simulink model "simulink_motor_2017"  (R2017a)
settings: Solver=VariableStepAuto  StartTime=0.0  StopTime=1  MaxStep=0.0001  RelTol=1e-5
undefined symbols (not defined in the file or in its folder): j

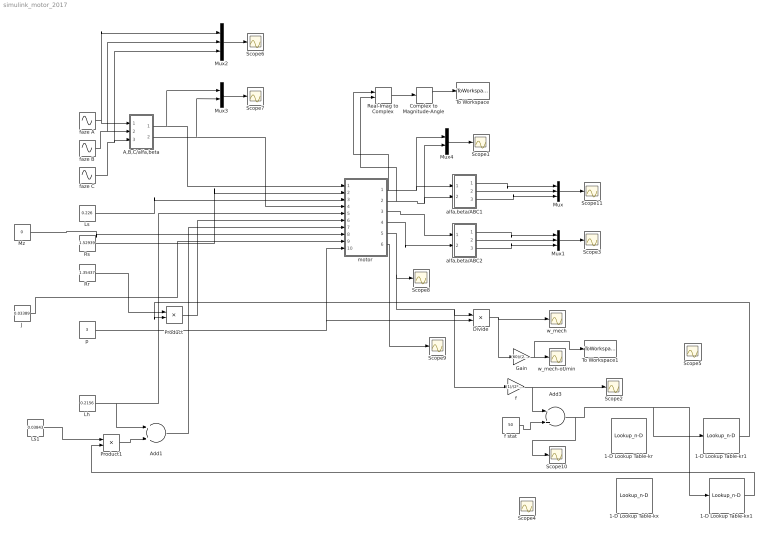
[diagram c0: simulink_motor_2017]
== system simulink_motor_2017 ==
  1-D Lookup Table-kr : Lookup_n-D  NumberOfTableDimensions=1  BreakpointsForDimension1="[0\t0.505050505050505\t1.01010101010101\t1.51515151515152\t2.02020202020202\t2.52525252525253\t3.03030303030303\t3.53535353535354\t4.04040404040404\t4.54545454545455\t5.05050505050505\t5.55555555555556\t6.06060606060606\t6.56565656565657\t7.07070707070707\t7.57575757575758\t8.08080808080808\t8.58585858585859\t9.09090909090909\t9.59595959595960\t10.1010101010101\t10.6060606060606\t11.1111111111111\t11.6161616161616\t12.12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"  Table="[1.00000000000000\t1.00008864994525\t1.00035453875263\t1.00079748344328\t1.00141717940610\t1.00221320092722\t1.00318500192865\t1.00433191691399\t1.00565316211802\t1.00714783685648\t1.00881492507177\t1.01065329706958\t1.01266171144098\t1.01483881716387\t1.01718315587736\t1.01969316432170\t1.02236717693666\t1.02520342860997\t1.02820005756793\t1.03135510839921\t1.03466653520308\t1.03813220485274\t1.04174990036446\t1.045517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"  InternalRulePriority=Speed  RndMeth=Simplest
  1-D Lookup Table-kr1 : Lookup_n-D  NumberOfTableDimensions=1  BreakpointsForDimension1="[0\t1.02040816326531\t2.04081632653061\t3.06122448979592\t4.08163265306123\t5.10204081632653\t6.12244897959184\t7.14285714285714\t8.16326530612245\t9.18367346938776\t10.2040816326531\t11.2244897959184\t12.2448979591837\t13.2653061224490\t14.2857142857143\t15.3061224489796\t16.3265306122449\t17.3469387755102\t18.3673469387755\t19.3877551020408\t20.4081632653061\t21.4285714285714\t22.4489795918367\t23.4693877551020\t24.489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"  Table="[1.00000000000000\t1.00077060964083\t1.00307777507260\t1.00690757634345\t1.01223704661737\t1.01903451494662\t1.02726007276191\t1.03686615140433\t1.04779819537135\t1.05999541393792\t1.07339159250137\t1.08791594439901\t1.10349398404126\t1.12004840293262\t1.13749993143670\t1.15576817087600\t1.17477238262788\t1.19443222316750\t1.21466841640173\t1.23540335703097\t1.25656164097697\t1.27807052105181\t1.29986028795912\t1.321864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"  InternalRulePriority=Speed  RndMeth=Simplest
  1-D Lookup Table-kx : Lookup_n-D  NumberOfTableDimensions=1  BreakpointsForDimension1="[0\t0.505050505050505\t1.01010101010101\t1.51515151515152\t2.02020202020202\t2.52525252525253\t3.03030303030303\t3.53535353535354\t4.04040404040404\t4.54545454545455\t5.05050505050505\t5.55555555555556\t6.06060606060606\t6.56565656565657\t7.07070707070707\t7.57575757575758\t8.08080808080808\t8.58585858585859\t9.09090909090909\t9.59595959595960\t10.1010101010101\t10.6060606060606\t11.1111111111111\t11.6161616161616\t12.12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"  Table="[1.04727985024947\t1.04725773631299\t1.04719140989840\t1.04708091716353\t1.04692633494882\t1.04672777064382\t1.04648536200084\t1.04619927689636\t1.04586971304107\t1.04549689763934\t1.04508108699933\t1.04462256609487\t1.04412164808060\t1.04357867376190\t1.04299401102106\t1.04236805420188\t1.04170122345412\t1.04099396404022\t1.04024674560607\t1.03946006141828\t1.03863442756993\t1.03777038215741\t1.03686848443050\t1.035929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"  InternalRulePriority=Speed  RndMeth=Simplest
  1-D Lookup Table-kx1 : Lookup_n-D  NumberOfTableDimensions=1  BreakpointsForDimension1="[0\t1.02040816326531\t2.04081632653061\t3.06122448979592\t4.08163265306123\t5.10204081632653\t6.12244897959184\t7.14285714285714\t8.16326530612245\t9.18367346938776\t10.2040816326531\t11.2244897959184\t12.2448979591837\t13.2653061224490\t14.2857142857143\t15.3061224489796\t16.3265306122449\t17.3469387755102\t18.3673469387755\t19.3877551020408\t20.4081632653061\t21.4285714285714\t22.4489795918367\t23.4693877551020\t24.489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"  Table="[1.00000000000000\t0.999555176608620\t0.998223403700545\t0.996012732286468\t0.992936445906495\t0.989012862377403\t0.984265063983984\t0.978720563445998\t0.972410914526099\t0.965371277307041\t0.957639948925946\t0.949257870899851\t0.940268124122870\t0.930715422193039\t0.920645612984507\t0.910105197377543\t0.899140872861085\t0.887799108398502\t0.876125755562974\t0.864165699565028\t0.851962552463579\t0.839558389616062\t0.82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"  InternalRulePriority=Speed  RndMeth=Simplest
  A,B,C/alfa,beta : Subsystem
  Add1 : Sum
  Add3 : Sum  Inputs=-+
  Complex to Magnitude-Angle : ComplexToMagnitudeAngle
  Divide : Product  Inputs=*/
  Gain : Gain  Gain=(60)/(2*pi)
  J : Constant  Value=0.03389
  Lh : Constant  Value=0.2156
  Ls : Constant  Value=0.226
  Ls1 : Constant  Value=0.03843
  Mux : Mux  Inputs=3
  Mux1 : Mux  Inputs=3
  Mux2 : Mux  Inputs=3
  Mux3 : Mux  Inputs=2
  Mux4 : Mux  Inputs=2
  Mz : Constant  Value=0
  Product : Product
  Product1 : Product
  Real-Imag to Complex : RealImagToComplex
  Rr : Constant  Value=1.35437
  Rs : Constant  Value=1.52939
  Scope{1..11} (11 alike) : Scope
  To Workspace : ToWorkspace  VariableName=Istat  SampleTime=-1
  To Workspace1 : ToWorkspace  VariableName=ot  SampleTime=-1
  alfa,beta/ABC1 : Subsystem
  alfa,beta/ABC2 : Subsystem
  f : Gain  Gain=(1)/(2*pi)
  f stat : Constant  Value=50
  faze A : Sin  Amplitude=230*1.41421356237309  Frequency=314.159265  SampleTime=0
  faze B : Sin  Amplitude=230*1.41421356237309  Frequency=314.159265  Phase=-(2*pi/3)  SampleTime=0
  faze C : Sin  Amplitude=230*1.41421356237309  Frequency=314.159265  Phase=(2*pi/3)  SampleTime=0
  motor : Subsystem
  p : Constant  Value=3
  w_mech : Scope
  w_mech-ot/min : Scope
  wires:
  faze A/1 -> Mux2/1, A,B,C/alfa,beta/1(In1)
  faze B/1 -> Mux2/2, A,B,C/alfa,beta/2(In2)
  faze C/1 -> Mux2/3, A,B,C/alfa,beta/3(In3)
  A,B,C/alfa,beta/1(Out1) -> Mux3/1, motor/1(Us_alfa)
  Rs/1 -> motor/2(Rs)
  Ls/1 -> motor/3(Ls)
  Lh/1 -> Add1/1, motor/5(Lh)
  motor/3(Ir_alfa1) -> alfa,beta/ABC2/1(Ir_alfa)
  motor/4(Ir_beta) -> alfa,beta/ABC2/2(Ir_beta)
  motor/1(Is_alfa) -> Real-Imag to Complex/1, Mux4/1, alfa,beta/ABC1/1(Is_alfa)
  motor/2(Is_beta) -> Real-Imag to Complex/2, Mux4/2, alfa,beta/ABC1/2(Is_beta)
  A,B,C/alfa,beta/2(Out2) -> Mux3/2, motor/4(Us beta)
  alfa,beta/ABC1/2(Out2) -> Mux/2
  alfa,beta/ABC1/3(Out3) -> Mux/3
  alfa,beta/ABC2/1(Out1) -> Mux1/1
  alfa,beta/ABC2/2(Out2) -> Mux1/2
  alfa,beta/ABC2/3(Out3) -> Mux1/3
  p/1 -> Divide/2, motor/10(p)
  Mz/1 -> motor/8(Mz)
  J/1 -> motor/9(J)
  motor/5(w_el) -> Scope8/1, f/1, Divide/1
  motor/6(M_elmag1) -> Scope9/1
  Divide/1 -> Gain/1, w_mech/1
  alfa,beta/ABC1/1(Out1) -> Mux/1
  Mux/1 -> Scope11/1
  Mux1/1 -> Scope3/1
  Mux2/1 -> Scope6/1
  Mux3/1 -> Scope7/1
  Mux4/1 -> Scope1/1
  Gain/1 -> To Workspace1/1, w_mech-ot/min/1
  f stat/1 -> Add3/2
  f/1 -> Scope2/1, Add3/1
  Add3/1 -> Scope10/1, 1-D Lookup Table-kr1/1, 1-D Lookup Table-kx1/1
  Rr/1 -> Product/1
  Product/1 -> motor/6(Rr)
  Real-Imag to Complex/1 -> Complex to Magnitude-Angle/1
  Complex to Magnitude-Angle/1 -> To Workspace/1
  1-D Lookup Table-kr1/1 -> Product/2
  1-D Lookup Table-kx1/1 -> Product1/2
  Add1/1 -> motor/7(Lr)
  Ls1/1 -> Product1/1
  Product1/1 -> Add1/2

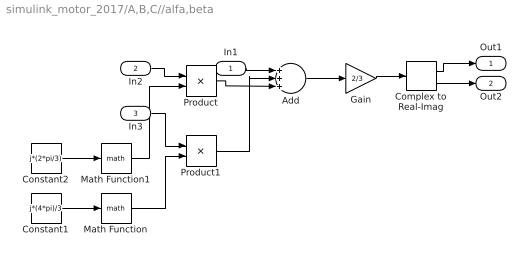
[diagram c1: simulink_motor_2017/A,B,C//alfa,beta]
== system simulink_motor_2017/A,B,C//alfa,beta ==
  In1 : Inport
  In2 : Inport  Port=2
  In3 : Inport  Port=3
  Add : Sum  Inputs=+++
  Complex to Real-Imag : ComplexToRealImag
  Constant1 : Constant  Value=j*(4*pi)/3
  Constant2 : Constant  Value=j*(2*pi/3)
  Gain : Gain  Gain=2/3
  Math Function : Math
  Math Function1 : Math
  Product : Product
  Product1 : Product
  Out1 : Outport
  Out2 : Outport  Port=2
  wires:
  Math Function/1 -> Product1/2
  Product1/1 -> Add/2
  Add/1 -> Gain/1
  Constant1/1 -> Math Function/1
  Product/1 -> Add/3
  Complex to Real-Imag/2 -> Out2/1
  Gain/1 -> Complex to Real-Imag/1
  Math Function1/1 -> Product/2
  In3/1 -> Product1/1
  Complex to Real-Imag/1 -> Out1/1
  Constant2/1 -> Math Function1/1
  In1/1 -> Add/1
  In2/1 -> Product/1

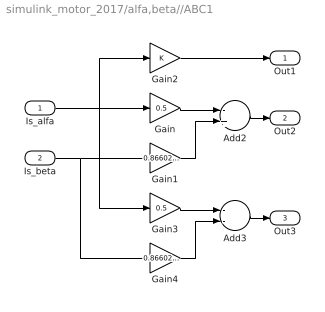
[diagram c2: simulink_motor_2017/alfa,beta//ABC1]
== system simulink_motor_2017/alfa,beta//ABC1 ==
  Is_alfa : Inport
  Is_beta : Inport  Port=2
  Add2 : Sum  Inputs=-+
  Add3 : Sum  Inputs=--
  Gain : Gain  Gain=0.5
  Gain1 : Gain  Gain=0.8660254037844
  Gain2 : Gain
  Gain3 : Gain  Gain=0.5
  Gain4 : Gain  Gain=0.8660254037844
  Out1 : Outport
  Out2 : Outport  Port=2
  Out3 : Outport  Port=3
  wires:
  Gain/1 -> Add2/1
  Is_alfa/1 -> Gain3/1, Gain2/1, Gain/1
  Gain4/1 -> Add3/2
  Gain1/1 -> Add2/2
  Is_beta/1 -> Gain4/1, Gain1/1
  Gain3/1 -> Add3/1
  Add2/1 -> Out2/1
  Add3/1 -> Out3/1
  Gain2/1 -> Out1/1

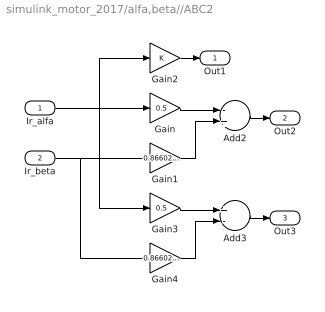
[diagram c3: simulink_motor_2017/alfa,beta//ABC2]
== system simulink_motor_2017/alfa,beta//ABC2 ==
  Ir_alfa : Inport
  Ir_beta : Inport  Port=2
  Add2 : Sum  Inputs=-+
  Add3 : Sum  Inputs=+-
  Gain : Gain  Gain=0.5
  Gain1 : Gain  Gain=0.8660254037844
  Gain2 : Gain
  Gain3 : Gain  Gain=0.5
  Gain4 : Gain  Gain=0.8660254037844
  Out1 : Outport
  Out2 : Outport  Port=2
  Out3 : Outport  Port=3
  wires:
  Gain/1 -> Add2/1
  Ir_alfa/1 -> Gain3/1, Gain2/1, Gain/1
  Gain4/1 -> Add3/2
  Gain1/1 -> Add2/2
  Ir_beta/1 -> Gain4/1, Gain1/1
  Gain3/1 -> Add3/1
  Add2/1 -> Out2/1
  Add3/1 -> Out3/1
  Gain2/1 -> Out1/1

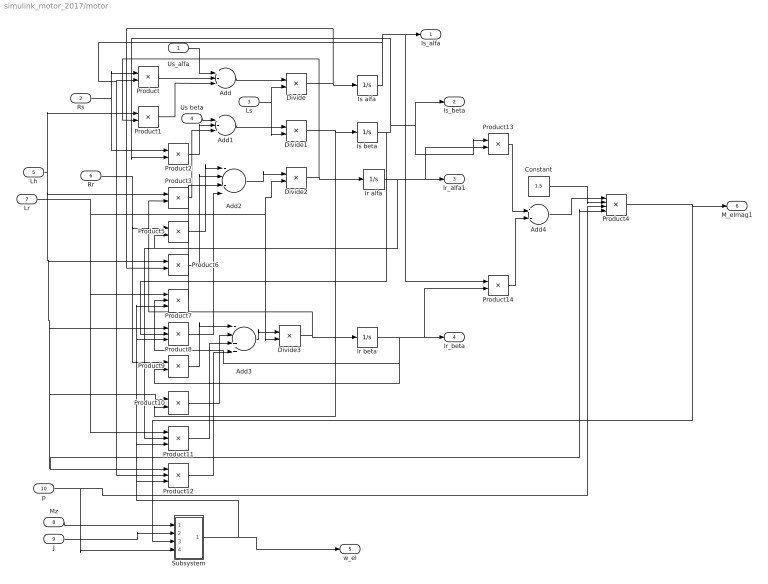
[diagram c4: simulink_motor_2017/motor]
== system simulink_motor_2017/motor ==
  Us_alfa : Inport
  Rs : Inport  Port=2
  Ls : Inport  Port=3
  Us beta : Inport  Port=4
  Lh : Inport  Port=5
  Rr : Inport  Port=6
  Lr : Inport  Port=7
  Mz : Inport  Port=8
  J : Inport  Port=9
  p : Inport  Port=10
  Add : Sum  Inputs=+--
  Add1 : Sum  Inputs=+--
  Add2 : Sum  Inputs=----
  Add3 : Sum  Inputs=--++
  Add4 : Sum  Inputs=+-
  Constant : Constant  Value=1.5
  Divide{,1..3} (4 alike) : Product  Inputs=*/
  Ir alfa : Integrator
  Ir beta : Integrator
  Is alfa : Integrator
  Is beta : Integrator
  Product{,1..3,5..6,9..10,13..14} (10 alike) : Product
  Product{7..8,11..12} (4 alike) : Product  Inputs=3
  Product4 : Product  Inputs=4
  Subsystem : Subsystem
  Is_alfa : Outport
  Is_beta : Outport  Port=2
  Ir_alfa1 : Outport  Port=3
  Ir_beta : Outport  Port=4
  w_el : Outport  Port=5
  M_elmag1 : Outport  Port=6
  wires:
  Lh/1 -> Product4/4, Product12/1, Product10/1, Product8/1, Product6/1, Product3/1, Product1/1
  Product6/1 -> Add2/2
  Product8/1 -> Add2/4
  Ir alfa/1 -> Product13/2, Ir_alfa1/1, Product11/2, Product5/2
  Product7/1 -> Add2/3
  Rs/1 -> Product2/1, Product/1
  Product1/1 -> Add/3
  Product/1 -> Add/2
  Is beta/1 -> Is_beta/1, Product13/1, Product2/2, Product8/2
  Ls/1 -> Divide1/2, Divide/2
  Add1/1 -> Divide1/1
  Divide2/1 -> Ir alfa/1, Product1/2
  Add/1 -> Divide/1
  Is alfa/1 -> Product14/1, Is_alfa/1, Product12/2, Product/2
  Product3/1 -> Add1/3
  Add2/1 -> Divide2/1
  Product5/1 -> Add2/1
  Rr/1 -> Product9/1, Product5/1
  Lr/1 -> Product11/1, Product7/1, Divide2/2, Divide3/2
  Product2/1 -> Add1/2
  Us beta/1 -> Add1/1
  Us_alfa/1 -> Add/1
  Product10/1 -> Add3/2
  Product11/1 -> Add3/3
  Divide3/1 -> Ir beta/1, Product3/2
  Product12/1 -> Add3/4
  Divide/1 -> Product6/2, Is alfa/1
  Divide1/1 -> Product10/2, Is beta/1
  Product9/1 -> Add3/1
  Add3/1 -> Divide3/1
  Mz/1 -> Subsystem/1(Mz)
  J/1 -> Subsystem/2(J)
  p/1 -> Subsystem/4(p), Product4/3
  Subsystem/1(Out1) -> Product12/3, Product11/3, Product8/3, Product7/3, w_el/1
  Ir beta/1 -> Product14/2, Ir_beta/1, Product9/2, Product7/2
  Product13/1 -> Add4/1
  Product14/1 -> Add4/2
  Add4/1 -> Product4/1
  Constant/1 -> Product4/2
  Product4/1 -> Subsystem/3(Melmag), M_elmag1/1

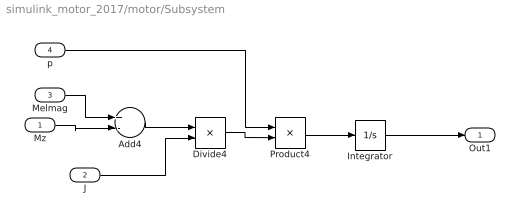
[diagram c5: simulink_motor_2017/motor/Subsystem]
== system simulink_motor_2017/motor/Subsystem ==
  Mz : Inport
  J : Inport  Port=2
  Melmag : Inport  Port=3
  p : Inport  Port=4
  Add4 : Sum  Inputs=+-
  Divide4 : Product  Inputs=*/
  Integrator : Integrator
  Product4 : Product
  Out1 : Outport
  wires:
  Melmag/1 -> Add4/1
  Add4/1 -> Divide4/1
  Integrator/1 -> Out1/1
  p/1 -> Product4/1
  Product4/1 -> Integrator/1
  J/1 -> Divide4/2
  Mz/1 -> Add4/2
  Divide4/1 -> Product4/2
